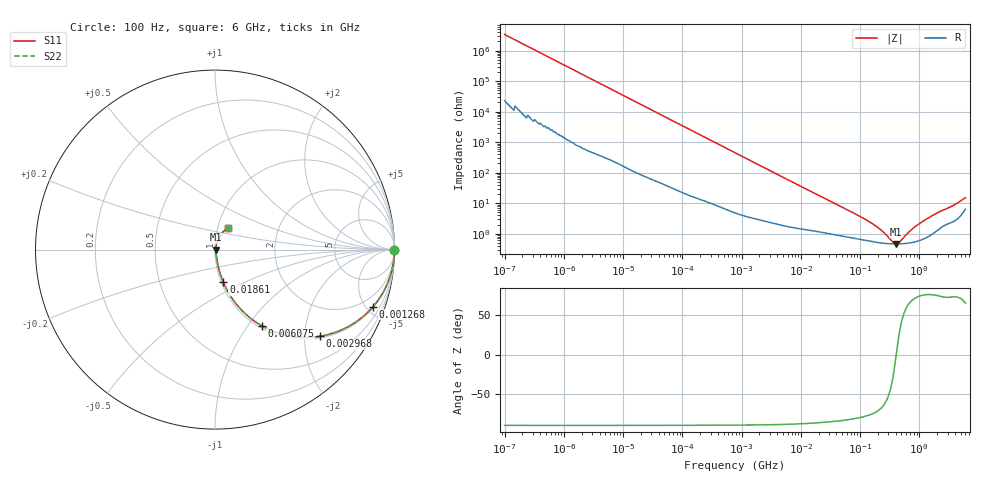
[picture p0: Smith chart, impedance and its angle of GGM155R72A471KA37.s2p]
!Murata Part Number: GGM155R72A471KA37
!These Parameters are Measured in Series Mode Connection
!Data Generated on Jun 19, 2026
!  o--ll--o
!Port1  Port2
!  o------o
!Operation Temp=25[degC], DC Bias Voltage=0[V]
!Freq. Start=100[Hz] Stop=6[GHz] 401[Steps]
# Hz S RI R 50
!Freq.(Hz) S11(Real) S11(Imag) S21(Real) S21(Imag) S12(Real) S12(Imag) S22(Real) S22(Imag)
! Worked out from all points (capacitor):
!   401 points, 100 Hz to 6 GHz, reference 50 ohm
!   read as one part in series: C = 470 pF near 109 Hz
!   lowest |Z| = 462 mohm at 408.7 MHz (marker M1)
!   series resonance near 408.3 MHz, so ESL is about 320 pH
!   S11 on the Smith chart (normalised r, x): 100 Hz: open; 1.268 MHz: 1.07, -5.51; 2.968 MHz: 1.05, -2.37; 6.075 MHz: 1.03, -1.16; 18.61 MHz: 1.02, -0.39; 6 GHz: 1.13, +0.27
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100  1 -2.95e-05  2e-07 2.95e-05  2e-07 2.95e-05  1 -2.95e-05
350  1 -0.000103  5e-07 0.000103  5e-07 0.000103  1 -0.000103
2008  1 -0.000588  2.6e-06 0.000588  2.6e-06 0.000588  1 -0.000588
40335  0.9998 -0.0117  0.000203 0.0117  0.000203 0.0117  0.9998 -0.0117
241822  0.9946 -0.0694  0.0054 0.0694  0.0054 0.0694  0.9946 -0.0694
774597  0.9509 -0.2107  0.0491 0.2107  0.0491 0.2107  0.9509 -0.2107
1267578  0.8806 -0.3178  0.1194 0.3178  0.1194 0.3178  0.8806 -0.3178
2967816  0.5824 -0.4833  0.4176 0.4833  0.4176 0.4833  0.5824 -0.4833
6075234  0.2596 -0.4241  0.7404 0.4241  0.7404 0.4241  0.2596 -0.4241
9506416  0.1322 -0.3199  0.8678 0.3199  0.8678 0.3199  0.1322 -0.3199
1.555665e7  0.0609 -0.2135  0.9391 0.2135  0.9391 0.2135  0.0609 -0.2135
1.86079e7  0.0465 -0.182  0.9535 0.182  0.9535 0.182  0.0465 -0.182
4.35672e7  0.0155 -0.0819  0.9845 0.0819  0.9845 0.0819  0.0155 -0.0819
1.395531e8  0.00633 -0.0245  0.9937 0.0245  0.9937 0.0245  0.00633 -0.0245
2.183701e8  0.00515 -0.0129  0.9949 0.0129  0.9949 0.0129  0.00515 -0.0129
3.124326e8  0.00469 -0.0053  0.9953 0.0053  0.9953 0.0053  0.00469 -0.0053
3.737127e8  0.0046 -0.00174  0.9954 0.00174  0.9954 0.00174  0.0046 -0.00174
4.087225e8  0.0046 2.09e-05  0.9954 -2.09e-05  0.9954 -2.09e-05  0.0046 2.09e-05
4.674818e8  0.00462 0.00268  0.9954 -0.00268  0.9954 -0.00268  0.00462 0.00268
7.31507e8  0.0052 0.0122  0.9948 -0.0122  0.9948 -0.0122  0.0052 0.0122
1.144649e9  0.00707 0.0242  0.9929 -0.0242  0.9929 -0.0242  0.00707 0.0242
6e9  0.0752 0.1194  0.9248 -0.1194  0.9248 -0.1194  0.0752 0.1194
